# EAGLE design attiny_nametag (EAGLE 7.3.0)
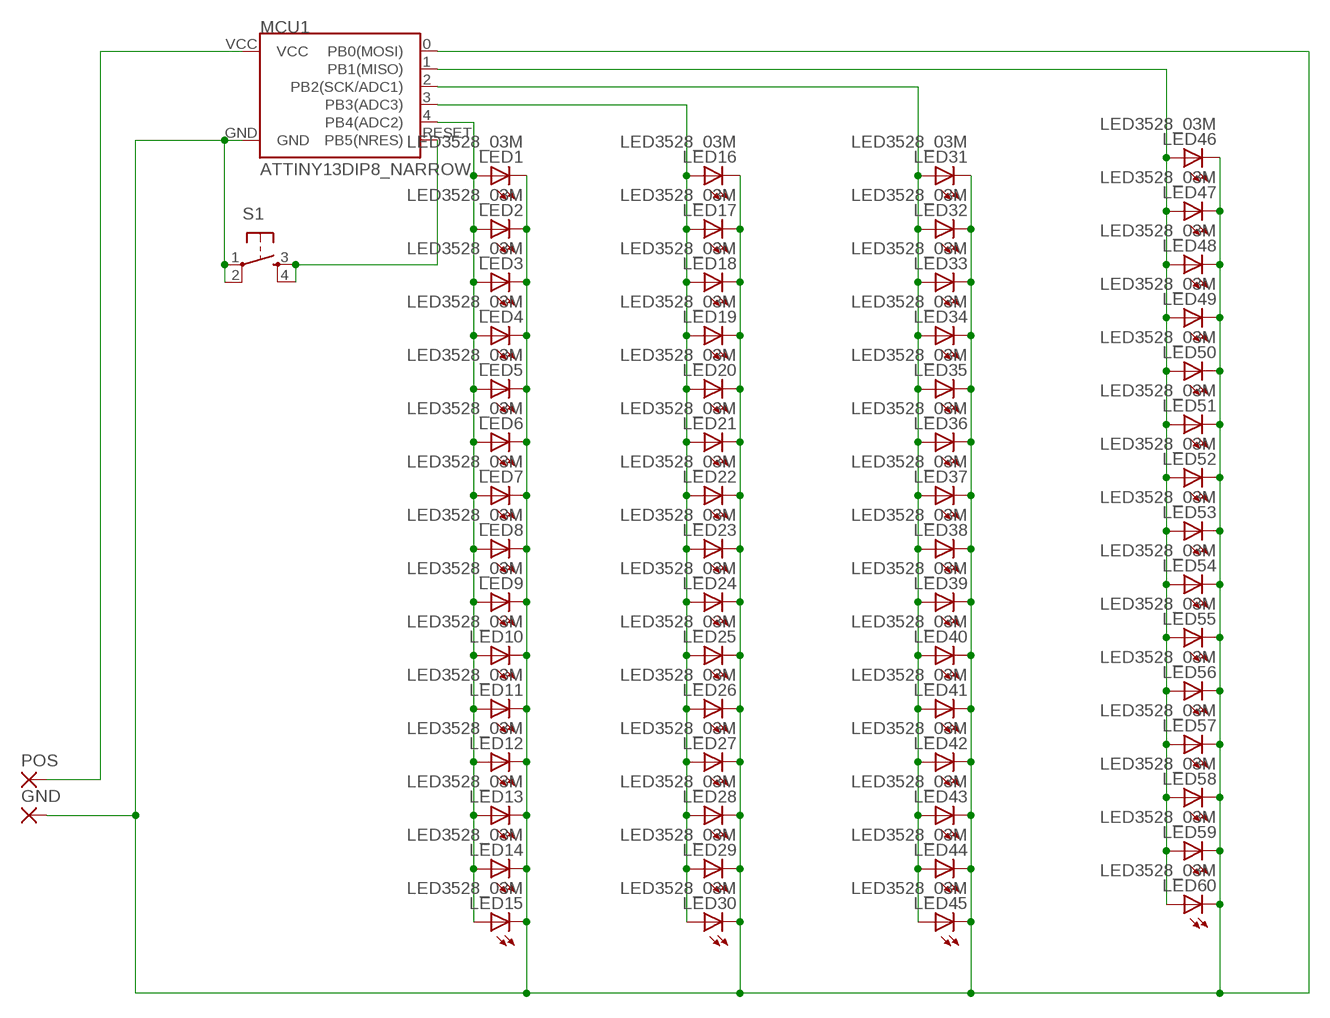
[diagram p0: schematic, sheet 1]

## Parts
GND  SMD5  [SMD2,54-5,08]
LED1  LED3528_03M  [LED3528_03M]
LED2  LED3528_03M  [LED3528_03M]
LED3  LED3528_03M  [LED3528_03M]
LED4  LED3528_03M  [LED3528_03M]
LED5  LED3528_03M  [LED3528_03M]
LED6  LED3528_03M  [LED3528_03M]
LED7  LED3528_03M  [LED3528_03M]
LED8  LED3528_03M  [LED3528_03M]
LED9  LED3528_03M  [LED3528_03M]
LED10  LED3528_03M  [LED3528_03M]
LED11  LED3528_03M  [LED3528_03M]
LED12  LED3528_03M  [LED3528_03M]
LED13  LED3528_03M  [LED3528_03M]
LED14  LED3528_03M  [LED3528_03M]
LED15  LED3528_03M  [LED3528_03M]
LED16  LED3528_03M  [LED3528_03M]
LED17  LED3528_03M  [LED3528_03M]
LED18  LED3528_03M  [LED3528_03M]
LED19  LED3528_03M  [LED3528_03M]
LED20  LED3528_03M  [LED3528_03M]
LED21  LED3528_03M  [LED3528_03M]
LED22  LED3528_03M  [LED3528_03M]
LED23  LED3528_03M  [LED3528_03M]
LED24  LED3528_03M  [LED3528_03M]
LED25  LED3528_03M  [LED3528_03M]
LED26  LED3528_03M  [LED3528_03M]
LED27  LED3528_03M  [LED3528_03M]
LED28  LED3528_03M  [LED3528_03M]
LED29  LED3528_03M  [LED3528_03M]
LED30  LED3528_03M  [LED3528_03M]
LED31  LED3528_03M  [LED3528_03M]
LED32  LED3528_03M  [LED3528_03M]
LED33  LED3528_03M  [LED3528_03M]
LED34  LED3528_03M  [LED3528_03M]
LED35  LED3528_03M  [LED3528_03M]
LED36  LED3528_03M  [LED3528_03M]
LED37  LED3528_03M  [LED3528_03M]
LED38  LED3528_03M  [LED3528_03M]
LED39  LED3528_03M  [LED3528_03M]
LED40  LED3528_03M  [LED3528_03M]
LED41  LED3528_03M  [LED3528_03M]
LED42  LED3528_03M  [LED3528_03M]
LED43  LED3528_03M  [LED3528_03M]
LED44  LED3528_03M  [LED3528_03M]
LED45  LED3528_03M  [LED3528_03M]
LED46  LED3528_03M  [LED3528_03M]
LED47  LED3528_03M  [LED3528_03M]
LED48  LED3528_03M  [LED3528_03M]
LED49  LED3528_03M  [LED3528_03M]
LED50  LED3528_03M  [LED3528_03M]
LED51  LED3528_03M  [LED3528_03M]
LED52  LED3528_03M  [LED3528_03M]
LED53  LED3528_03M  [LED3528_03M]
LED54  LED3528_03M  [LED3528_03M]
LED55  LED3528_03M  [LED3528_03M]
LED56  LED3528_03M  [LED3528_03M]
LED57  LED3528_03M  [LED3528_03M]
LED58  LED3528_03M  [LED3528_03M]
LED59  LED3528_03M  [LED3528_03M]
LED60  LED3528_03M  [LED3528_03M]
MCU1  ATTINY13DIP8_NARROW  [DIP8_NARROW]
POS  SMD5  [SMD2,54-5,08]
S1  TAC_SWITCHPTH  [TACTILE-PTH]

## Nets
N$3: MCU1.VCC POS.1(P)
N$4: LED1.A LED2.A LED3.A LED4.A LED5.A LED6.A LED7.A LED8.A LED9.A LED10.A LED11.A LED12.A LED13.A LED14.A LED15.A MCU1.4(PB4(ADC2))
N$6: LED31.A LED32.A LED33.A LED34.A LED35.A LED36.A LED37.A LED38.A LED39.A LED40.A LED41.A LED42.A LED43.A LED44.A LED45.A MCU1.2(PB2(SCK/ADC1))
N$7: LED16.A LED17.A LED18.A LED19.A LED20.A LED21.A LED22.A LED23.A LED24.A LED25.A LED26.A LED27.A LED28.A LED29.A LED30.A MCU1.3(PB3(ADC3))
N$9: LED46.A LED47.A LED48.A LED49.A LED50.A LED51.A LED52.A LED53.A LED54.A LED55.A LED56.A LED57.A LED58.A LED59.A LED60.A MCU1.1(PB1(MISO))
N$14: GND.1(P) LED1.C LED2.C LED3.C LED4.C LED5.C LED6.C LED7.C LED8.C LED9.C LED10.C LED11.C LED12.C LED13.C LED14.C LED15.C LED16.C LED17.C LED18.C LED19.C LED20.C LED21.C LED22.C LED23.C LED24.C LED25.C LED26.C LED27.C LED28.C LED29.C LED30.C LED31.C LED32.C LED33.C LED34.C LED35.C LED36.C LED37.C LED38.C LED39.C LED40.C LED41.C LED42.C LED43.C LED44.C LED45.C LED46.C LED47.C LED48.C LED49.C LED50.C LED51.C LED52.C LED53.C LED54.C LED55.C LED56.C LED57.C LED58.C LED59.C LED60.C MCU1.0(PB0(MOSI)) MCU1.GND S1.1 S1.2
N$21: MCU1.RESET(PB5(NRES)) S1.3 S1.4

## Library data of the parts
GND POS = wirepad:SMD5: SMD PAD
LED1-LED60 = name_tag:LED3528_03M: moved pads out 0.3mm
MCU1 = wiley:ATTINY13
S1 = SparkFun-Retired:TAC_SWITCH: Momentary Switch Button commonly used for reset or general input. Spark Fun Electronics SKU : COM-00097 SMT- SWCH-08247

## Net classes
0 default: width 0.8 mm, drill 0.8 mm, clearance 0.8 mm

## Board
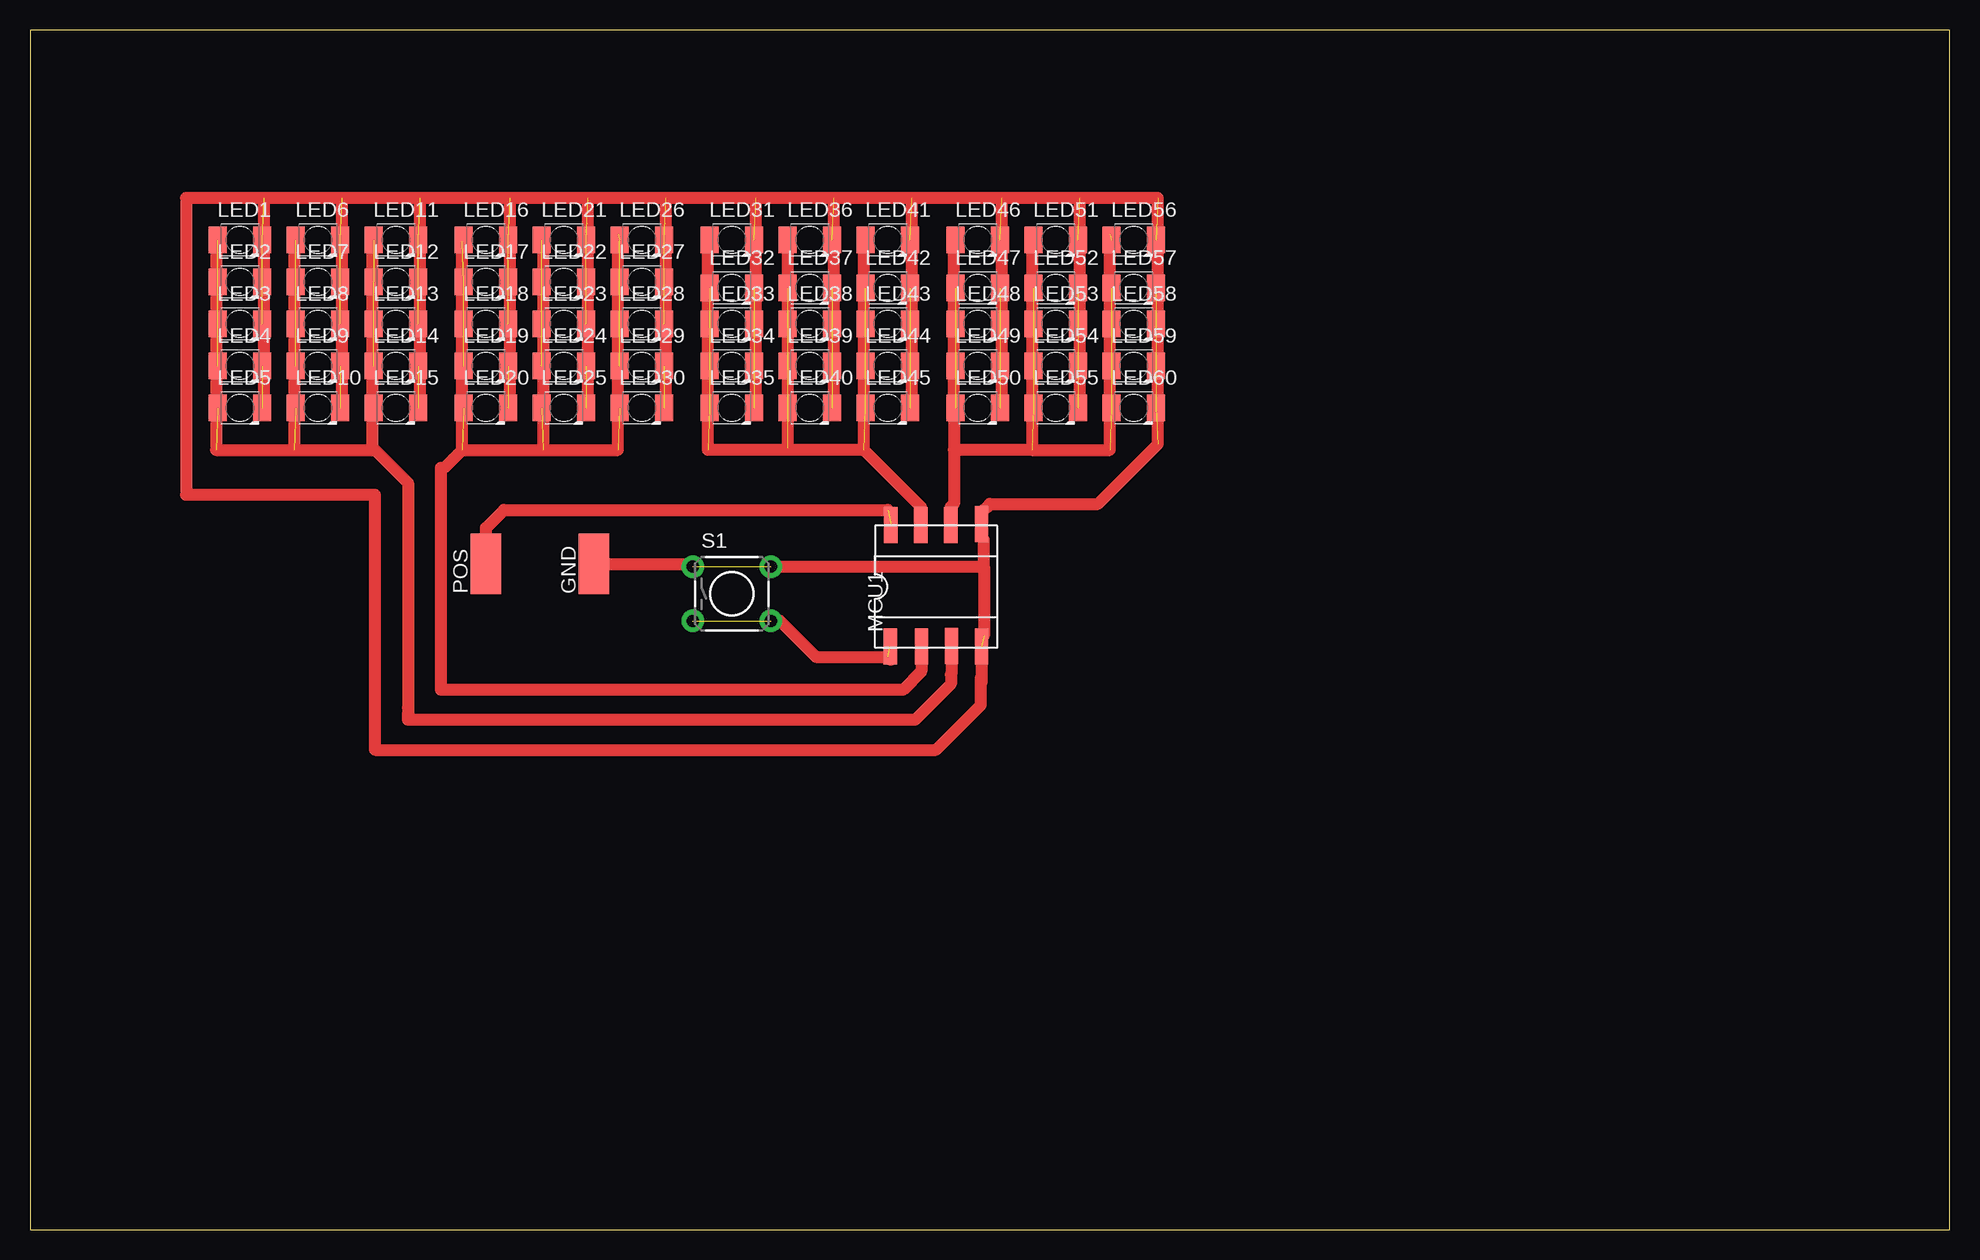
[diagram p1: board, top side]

Size 160 x 100 mm. Coordinates in mm from the lower left corner, seen from the top.
Outline: 0,0 160,0 160,100 0,100 0,0
Copper layers (1*16): Top 0.035mm / dielectric 1.5mm / Bottom 0.035mm
Design rules "default": minimum track width 10mil, minimum drill 24mil, track to track 8mil, track to pad 8mil, pad to pad 8mil, via to via 8mil, smd to smd 8mil, copper to edge 40mil, drill to drill 8mil, minimum pad ring 10mil, minimum via ring 8mil, stop-mask expansion 4mil, vias tented up to drill 0mil, thermal gap 10mil

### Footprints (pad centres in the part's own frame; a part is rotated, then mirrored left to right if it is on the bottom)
SMD2,54-5,08 = smd 2.54 x 5.08: 1 0,0
LED3528_03M = smd 1.5 x 2.2: A -1.85,0; C 1.85,0
DIP8_NARROW = smd 1.1 x 3: 0 5.8,5.8; 1 3.25,5.75; 2 0.75,5.75; 3 0.8,-4.4; 4 3.3,-4.35; GND 5.8,-4.4; RESET -1.8,-4.4; VCC -1.75,5.75
TACTILE-PTH = drill 1.016 pad 1.88: 1 -3.251,2.261; 2 3.251,2.261; 3 -3.251,-2.261; 4 3.251,-2.261

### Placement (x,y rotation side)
GND  47,55.5 0 top
LED1  17.5,82.5 0 top
LED2  17.5,79 0 top
LED3  17.5,75.5 0 top
LED4  17.5,72 0 top
LED5  17.5,68.5 0 top
LED6  24,82.5 0 top
LED7  24,79 0 top
LED8  24,75.5 0 top
LED9  24,72 0 top
LED10  24,68.5 0 top
LED11  30.5,82.5 0 top
LED12  30.5,79 0 top
LED13  30.5,75.5 0 top
LED14  30.5,72 0 top
LED15  30.5,68.5 0 top
LED16  38,82.5 0 top
LED17  38,79 0 top
LED18  38,75.5 0 top
LED19  38,72 0 top
LED20  38,68.5 0 top
LED21  44.5,82.5 0 top
LED22  44.5,79 0 top
LED23  44.5,75.5 0 top
LED24  44.5,72 0 top
LED25  44.5,68.5 0 top
LED26  51,82.5 0 top
LED27  51,79 0 top
LED28  51,75.5 0 top
LED29  51,72 0 top
LED30  51,68.5 0 top
LED31  58.5,82.5 0 top
LED32  58.5,78.5 0 top
LED33  58.5,75.5 0 top
LED34  58.5,72 0 top
LED35  58.5,68.5 0 top
LED36  65,82.5 0 top
LED37  65,78.5 0 top
LED38  65,75.5 0 top
LED39  65,72 0 top
LED40  65,68.5 0 top
LED41  71.5,82.5 0 top
LED42  71.5,78.5 0 top
LED43  71.5,75.5 0 top
LED44  71.5,72 0 top
LED45  71.5,68.5 0 top
LED46  79,82.5 0 top
LED47  79,78.5 0 top
LED48  79,75.5 0 top
LED49  79,72 0 top
LED50  79,68.5 0 top
LED51  85.5,82.5 0 top
LED52  85.5,78.5 0 top
LED53  85.5,75.5 0 top
LED54  85.5,72 0 top
LED55  85.5,68.5 0 top
LED56  92,82.5 0 top
LED57  92,78.5 0 top
LED58  92,75.5 0 top
LED59  92,72 0 top
LED60  92,68.5 0 top
MCU1  73.5,53 0 top
POS  38,55.5 0 top
S1  58.5,53 0 top

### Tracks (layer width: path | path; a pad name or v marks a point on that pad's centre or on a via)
N$3  (1 unrouted)
  Top 1: POS.1 38,58.5 39.5,60 71.5,60
N$4  (11 unrouted)
  Top 1: MCU1.4 76.8,46.3 76.75,46.25 76.75,45.5 73.75,42.5 31.5,42.5 31.5,43 31.5,43.5 31.5,62.25 28.75,65 28.5,65 | LED11.A 28.5,82.5 28.5,68.5 | 28.5,68.5 28.5,65 | LED15.A 28.5,68.5 | LED6.A 22,82.5 22,65 | 22,65 28.5,65 | LED1.A 15.5,82.5 15.5,65 22,65
N$6  (12 unrouted)
  Top 1: MCU1.2 74.25,60.25 69.5,65 | 69.5,65 69.5,82.35 LED41.A | 69.5,65 63,65 | 63,65 56.5,65 56.5,82.35 LED31.A | LED36.A 63.15,65.15 63,65
N$7  (13 unrouted)
  Top 1: MCU1.3 74.3,46.55 72.75,45 34.25,45 34.25,63.5 34.5,63.5 36,65 | 36,65 36,82.35 LED16.A | 36,65 42.75,65 | 42.75,65 49,65 49,83 | LED21.A 42.75,82.5 42.75,65
N$9  (12 unrouted)
  Top 1: MCU1.1 76.75,60.25 77,60.5 77,65 | 77,68.5 77,82.35 LED46.A | LED50.A 77,68.5 | 77,68.5 77,65 | LED51.A 83.5,82.5 83.5,65 | 83.5,65 77,65 | 83.5,65 90,65 90,83
N$14  (51 unrouted)
  Top 1: GND.1 55.01,55.5 S1.1 | S1.2 79.5,55.26 | 79.5,55.26 79.5,57.5 | 79.5,55.26 79.5,49.5 | MCU1.0 79.3,59.8 80,60.5 89,60.5 94,65.5 94,86 87.5,86 | 87.5,86 81,86 | 81,86 73.5,86 | 73.5,86 67,86 | 67,86 60.5,86 | 60.5,86 53,86 | 53,86 46.5,86 | 46.5,86 40,86 | 40,86 32.5,86 | 32.5,86 26,86 | 26,86 19.5,86 | 19.5,86 13,86 13,61.25 28.75,61.25 28.75,40 75.5,40 79.25,43.75 79.25,45.95 79.3,46 | MCU1.GND 79.3,46 | 79.3,46 79.3,45.55 | LED5.C 19.5,68.5 19.5,86 | LED10.C 26,68.5 26,86 | LED15.C 32.5,68.5 32.5,86 | LED20.C 40,68.5 40,86 | LED25.C 46.5,68.5 46.5,86 | LED30.C 53,68.5 53,86 | LED35.C 60.5,68.5 60.5,86 | LED40.C 67,68.5 67,86 | LED50.C 81,68.5 81,86 | LED55.C 87.5,68.5 87.5,86 | LED45.C 73.5,68.5 73.5,86
N$21  (2 unrouted)
  Top 1: S1.4 62.51,50.74 65.5,47.75 71.5,47.75 71.75,47.5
